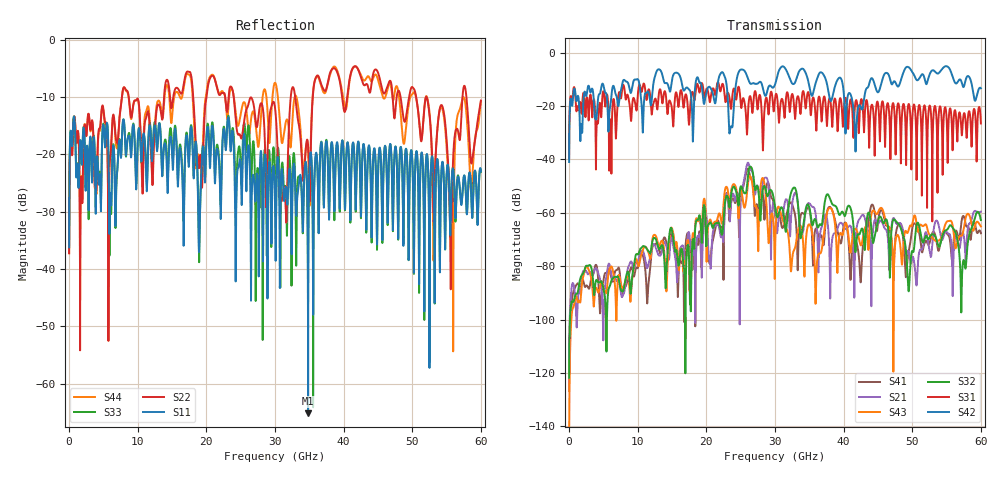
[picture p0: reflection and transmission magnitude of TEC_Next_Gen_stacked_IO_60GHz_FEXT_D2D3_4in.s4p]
!! CHANNEL DESCRIPTION:  Next Generation 28Gbps Press-fit Stacked I/O Connector
!!  with 4" 5-6-5 Megtron 6 Stripline trace on host side and 1.25" 7-5-7 Megtron 6 Microstrip trace on plug side
!! HOST PCB DESCRIPTION:  PCB thickness 3.425 mm
!!  26 Layer Board, 15 GND planes, 4 Layer route-out on Layers 7,11,17,21, 8mil stub on vias
!!  Pairs on following layers
!!  Layer 07 - A02A03 A14A15 D05D06
!!  Layer 11 - D020D3 C05C06 D14D15
!!  Layer 17 - C02C03 B05B06 C14C15
!!  Layer 21 - B02B03 A05A06 B14B15
!! CONNECTOR DESCRIPTION:  Next Generation 28Gbps Press-fit Stacked I/O Connector
!! PLUG-IN CARD DESCRIPTION:  PCB thickness 1mm thick
!!  6 Layer Board, 4 GND planes, 0.35 x 1.4mm mating pads
!!  Micro-strip diff traces referenced to GND plane 3mils down, 2nd GND plane 17mils from top of board
!!  PCB GND planes are symmetric
!! MODEL DESCRIPTION: TE Connectivity S-parameter model produced from Macro-model, Extracted .s4p FEXT (Victim B05B06 - Aggressor D02D03)
!! MODEL DATE: 5/15/2014 CR32f, FPR23
!! MODEL STATUS: Developmental
!! MODEL GEOMETRY: 4 Rows - Rows A, B, C, D. 3 pairs in each row, 12 total pairs
!! MODEL FREQUENCY RANGE: DC to 60 GHz in 10 MHz frequency steps
!! MODEL EDGE RATE LIMITATION: 8.33 ps (Using conservative 0.5/Fmax rule of thumb)
!! TIME-DOMAIN TRANSFORM CAUTIONS:
!! 1.) Do not simulate transient edge rates faster than the number listed above.  Edge
!!  rates faster than this number contain significant spectral content at frequencies
!!  above the model's highest frequency.
!! 2.) Even when simulating edge rates that are slower than the number listed above, be
!!  aware that the best time resolution possible with a direct iFFT is (1 / 2Fmax).
!!  As a result, time resolution is typically not adequate for most time-domain
!!  simulations unless tricks such as frequency-domain zero-padding and windowing are
!!  used to minimize leakage and aliasing.
!! 3.) Because the model has a uniform frequency step, a direct iFFT will result in an
!!  impulse that that has a time length given by either (1 / Fstep) or (1 / 2Fstep),
!!  depending on the transform being used.  Care has been taken in selecting the
!!  frequency step to ensure a settled impulse response for the model.  Therefore,
!!  convolution with the model's impulse response should present no issues.  However,
!!  if directly concatenating s-parameter models in the frequency domain a user must
!!  either interpolate necessary interim frequencies or complete impulse response
!!  zero-padding.  Impulse response zero-padding is more difficult, but more accurate.
!! PORT DEFINITIONS:
!! Port  1  ----->  Host D02		B05 Module <-----  Port  2
!! Port  3  ----->  Host D03		B06 Module <-----  Port  4
! Touchstone data
! Created: 29-Sep-2014 by IdEM R2011 (7.0.3)
# Hz S MA R 50
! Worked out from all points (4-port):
!   6000 points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, 10 MHz to 60 GHz, reference 50 ohm
!   strongest paths, dB at 10 MHz, 15.01 GHz, 30.01 GHz, 45.01 GHz, 60 GHz:
!     S42: -41.0, -10.1, -12.0, -14.9, -13.4
!     S31: -39.6, -21.7, -17.2, -19.0, -26.6
!     S32: -121.8, -66.9, -57.7, -63.0, -62.7
!     S43: -145.0, -65.9, -75.5, -59.9, -65.1
!     S21: -119.3, -69.9, -58.6, -64.2, -59.6
!     S41: -126.7, -68.2, -60.7, -63.7, -67.7
!   lowest |S11| = -65.2 dB at 34.83 GHz (marker M1), VSWR 1.00, Z = 49.9 + j0.0189 ohm
!   |S11| at or under -10 dB: start of sweep to end of sweep
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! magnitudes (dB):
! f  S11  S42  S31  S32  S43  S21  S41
! 10 MHz  -36.2  -41.0  -39.6  -121.8  -145.0  -119.3  -126.7
! 20.54 GHz  -22.4  -13.0  -18.5  -63.6  -62.5  -78.6  -78.6
! 26.37 GHz  -24.1  -11.5  -16.3  -42.7  -46.3  -43.3  -46.3
! 34.83 GHz  -65.2  -10.5  -14.8  -57.0  -64.7  -56.5  -58.1
! 50.55 GHz  -19.8  -10.0  -28.9  -65.8  -62.7  -85.8  -64.5
! 55.58 GHz  -32.9  -6.9  -21.2  -64.7  -63.0  -69.2  -72.0
! 60 GHz  -23.0  -13.4  -26.6  -62.7  -65.1  -59.6  -67.7
